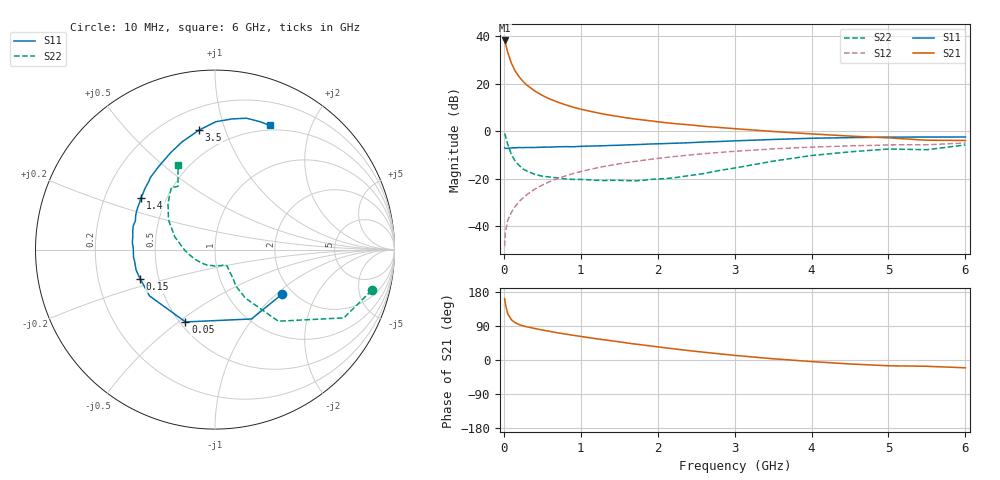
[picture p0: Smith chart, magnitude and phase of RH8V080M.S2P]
! SIEMENS Small Signal Semiconductors
! BFR106
! Si NPN RF Bipolar Junction Transistor in SOT23
! VCE = 8 V  IC = 80 mA
! Common Emitter S-Parameters:  August  1996
# GHz  S  MA  R  50
!  f  S11  S21  S12  S22
! GHz  MAG  ANG  MAG  ANG  MAG  ANG  MAG  ANG
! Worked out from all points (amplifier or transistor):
!   36 points, 10 MHz to 6 GHz, reference 50 ohm
!   highest |S21| = 38.2 dB at 10 MHz (marker M1)
!   |S21| within 3 dB of that: start of sweep to 35.03 MHz
!   unconditionally stable (mu >= 1): 215 MHz to 2.381 GHz
!   at 250 MHz: K = 1.04, MAG = 23.4 dB, |S12| = -28.1 dB
!   at 1.4 GHz: K = 1.07, MAG = 8.9 dB, |S12| = -14.3 dB
!   at 6 GHz: K = 0.98, MSG = 0.5 dB, |S12| = -5.0 dB
!   S11 on the Smith chart (normalised r, x): 10 MHz: 1.76, -1.09; 50 MHz: 0.53, -0.53; 150 MHz: 0.39, -0.16; 1.4 GHz: 0.36, +0.28; 3.5 GHz: 0.34, +0.82; 6 GHz: 0.45, +1.44
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0.01  0.4488 -33.5  81.72 161.7  0.0038 84.6  0.9018 -14.6
0.02  0.4366 -62.3  72.44 147.6  0.0074 71.4  0.8128 -27.9
0.05  0.4352 -112.2  46.24 122.1  0.0132 61.6  0.5327 -48.5
0.1  0.4469 -144.7  26.64 105.8  0.0198 62.7  0.318 -58.0
0.15  0.4473 -158.7  18.27 98.0  0.0264 66.5  0.2318 -60.2
0.2  0.4543 -165.5  13.94 93.5  0.033 69.2  0.1896 -57.9
0.25  0.4522 -171.1  11.17 90.0  0.0395 70.1  0.1598 -56.9
0.3  0.4561 -174.7  9.357 87.5  0.0464 71.6  0.1455 -56.6
0.4  0.4553 179.0  7.087 83.2  0.0601 72.6  0.1241 -54.6
0.5  0.462 175.2  5.681 79.1  0.0734 72.5  0.1131 -53.4
0.6  0.4642 170.7  4.756 75.4  0.0875 72.1  0.1087 -54.7
0.7  0.4706 166.9  4.114 71.7  0.1012 71.5  0.1042 -57.4
0.9  0.4713 160.2  3.22 65.3  0.1286 69.2  0.097 -60.7
1.1  0.487 153.6  2.686 59.1  0.1548 66.8  0.095 -69.9
1.4  0.5038 145.2  2.149 50.7  0.1935 62.9  0.0925 -83.5
1.7  0.5221 137.1  1.816 42.2  0.231 58.7  0.0902 -101.0
2.2  0.5577 124.7  1.46 29.7  0.2916 51.6  0.104 -133.2
2.8  0.6082 111.0  1.202 16.4  0.3575 42.7  0.149 -170.3
3.5  0.6717 97.6  0.989 3.3  0.4258 32.5  0.2347 162.5
4.5  0.7341 82.6  0.791 -10.5  0.4913 17.8  0.3684 135.3
5.5  0.7556 70.4  0.647 -16.6  0.5202 7.7  0.4086 120.4
6  0.756 66.2  0.64 -20.6  0.5651 0.8  0.5148 113.5
